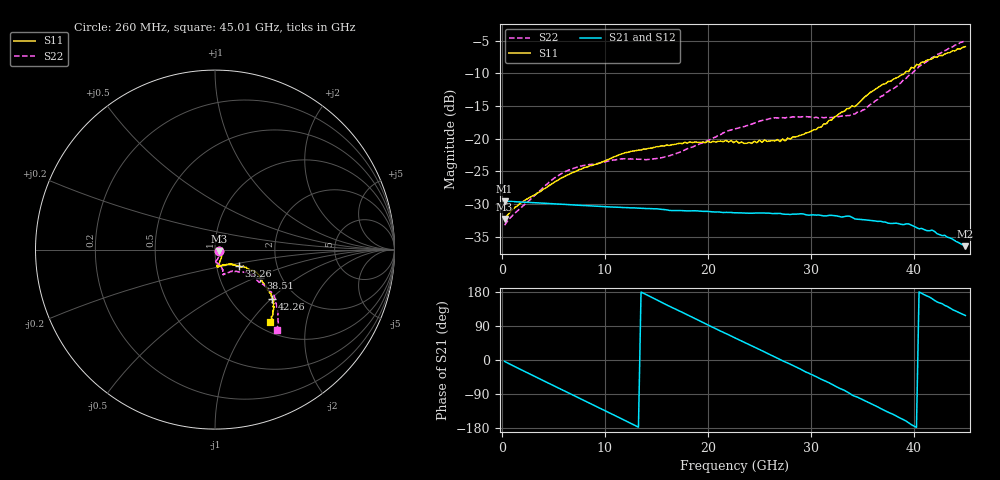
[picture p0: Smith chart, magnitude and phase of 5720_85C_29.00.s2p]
! Device:  ADRF5720
! Description: 0.5dB LSB GaAs MMIC 6-bit Digital Attenuator
! Frequency:  0.000009 -  40 GHz
! Ports:
!	RF1	= Port 1
!	RF2	= Port 2
! Vdd:  3.3 Volt
! Vss:  -3.3 Volt
! Control:  0/3.3 Volt
! State:  29.00 dB attenuation
! Data:  The device was measured using G-S-G Probes on a matrix board.
!  Data was collected using an calibrated 4 port network analyzer.
!  The reference plane for this measurement is at the launchers.
! Note:  Analog Devices supplies this data as a sample of measured data
!  for this product.  Your particular data for this product may vary.
!  Data was taken at 85 degrees C.
!  Analog Devices reserves the right to change this data at anytime.
# GHZ S DB R 45.0
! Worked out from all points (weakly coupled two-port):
!   180 points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, 260 MHz to 45.01 GHz, reference 45 ohm
!   highest |S21| = -29.57 dB at 260 MHz (marker M1); lowest = -36.5 dB at 45.01 GHz (marker M2)
!   lowest |S11| = -32.3 dB at 260 MHz (marker M3), VSWR 1.05, Z = 47.1 - j0.734 ohm
!   |S11| at or under -10 dB: start of sweep to 39.08 GHz
!   |S22| runs from -33.3 to -4.9 dB; largest |S21 - S12| = 0.00022
!   S11 on the Smith chart (normalised r, x): 260 MHz: 1.05, -0.02; 33.26 GHz: 1.28, -0.24; 38.51 GHz: 1.57, -0.54; 42.26 GHz: 1.51, -1.02; 45.01 GHz: 1.15, -1.25
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0.26  -32.28 -18.7  -29.57 -3.7  -29.56 -3.7  -33.26 -22.8
1.76  -29.93 -4.9  -29.69 -24.3  -29.68 -24.2  -30.70 -21.4
5.01  -26.74 -38.4  -29.98 -67.6  -29.96 -67.5  -26.12 -68.3
7.76  -24.64 -53.8  -30.22 -104.0  -30.21 -103.9  -24.16 -83.4
12.01  -22.12 -70.9  -30.56 -160.3  -30.54 -160.2  -23.06 -91.8
15.26  -21.20 -78.8  -30.79 155.5  -30.78 155.6  -22.96 -84.9
18.26  -20.49 -82.1  -31.06 116.1  -31.04 116.3  -21.38 -75.0
22.76  -20.35 -77.9  -31.35 56.7  -31.34 56.9  -18.44 -69.6
24.26  -20.72 -74.4  -31.42 37.7  -31.41 37.9  -17.75 -70.2
25.51  -20.19 -69.3  -31.39 21.2  -31.37 21.4  -17.06 -71.7
27.51  -20.34 -60.7  -31.58 -4.9  -31.57 -4.7  -16.81 -70.8
30.26  -18.64 -45.8  -31.67 -40.6  -31.65 -40.4  -16.80 -70.2
33.26  -15.79 -34.4  -31.93 -80.1  -31.93 -79.9  -16.52 -56.7
34.76  -14.39 -31.3  -32.36 -101.3  -32.35 -100.9  -15.95 -48.8
35.76  -12.91 -29.9  -32.52 -114.3  -32.51 -113.9  -14.77 -43.3
37.76  -11.19 -29.5  -32.99 -140.8  -33.00 -140.4  -12.47 -34.6
38.51  -10.53 -31.7  -33.01 -151.3  -33.00 -151.0  -11.72 -34.2
40.26  -8.62 -37.0  -33.61 -177.8  -33.59 -177.6  -9.40 -36.0
41.76  -7.77 -39.8  -34.01 162.2  -33.99 162.5  -7.57 -37.9
42.26  -7.52 -41.2  -34.56 153.4  -34.50 153.8  -7.09 -39.8
43.51  -6.79 -43.9  -35.20 137.2  -35.14 137.6  -6.03 -45.4
45.01  -5.89 -53.0  -36.47 117.4  -36.44 117.6  -4.94 -52.2
